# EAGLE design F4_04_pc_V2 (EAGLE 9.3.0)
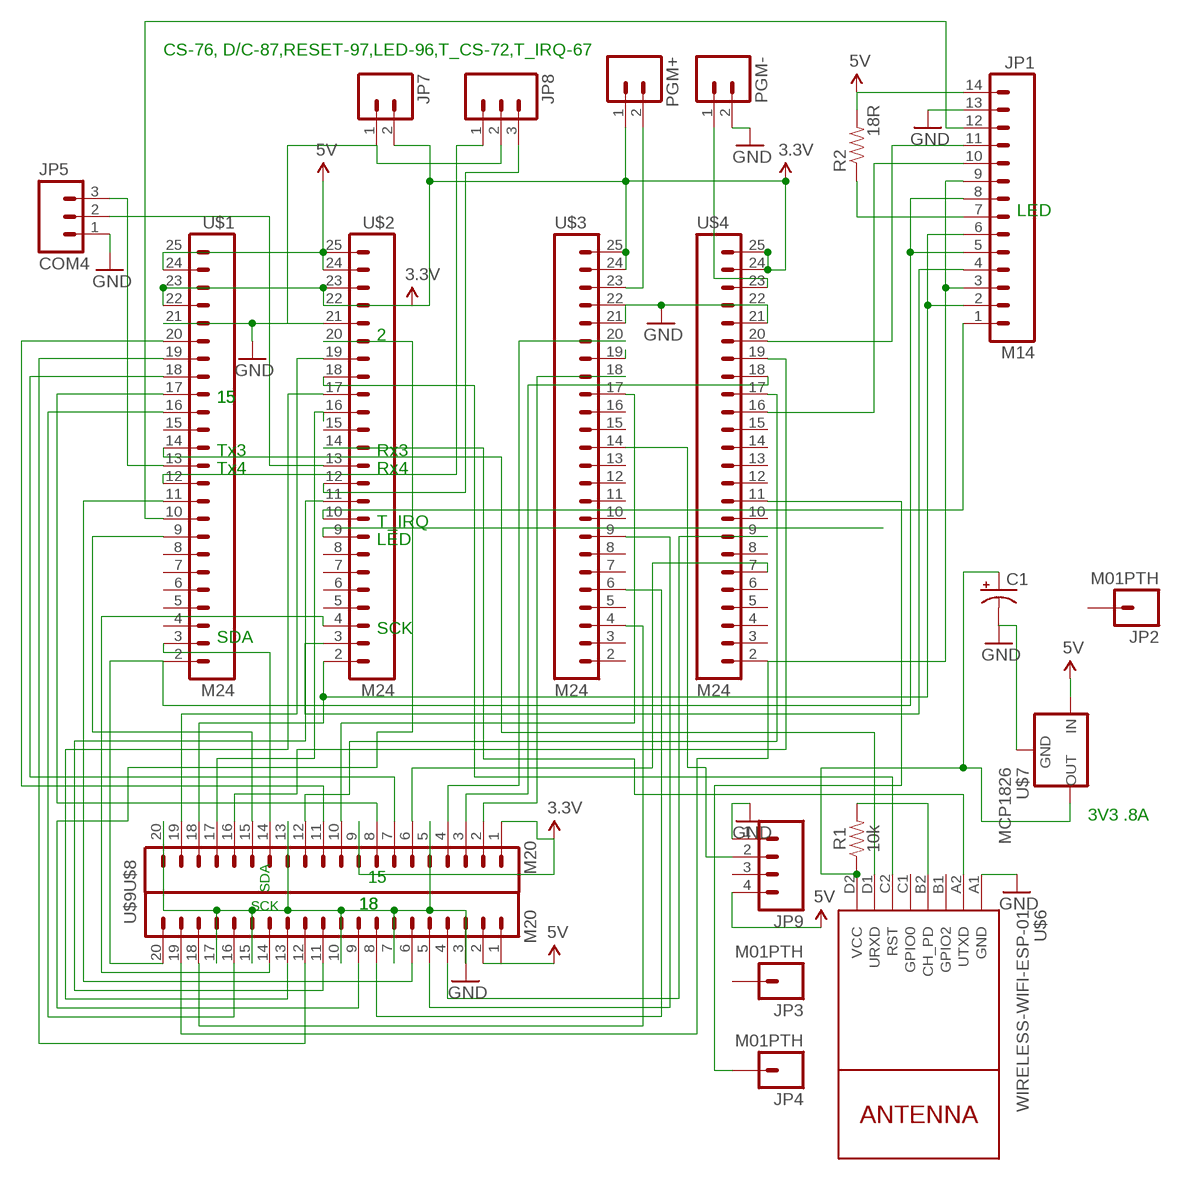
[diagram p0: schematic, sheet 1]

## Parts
C1  CAP_POLD  [PANASONIC_D]
JP1  M14  [1X14]
JP2  M01PTH  [1X01]
JP3  M01PTH  [1X01]
JP4  M01PTH  [1X01]
JP5  COM4  M03PTH  [1X03]
JP7  M02PTH  [1X02]
JP8  M03PTH  [1X03]
JP9  M04LOCK  [1X04_LOCK]
PGM+  M02PTH  [1X02]
PGM-  M02PTH  [1X02]
R1  10k  1KOHM-VERT-1/4W-1%  [AXIAL-0.1]
R2  18R  RESISTORPTH-1/6W  [1/6W-RES]
U$1  M24  [1X24]
U$2  M24  [1X24]
U$3  M24  [1X24]
U$4  M24  [1X24]
U$6  WIRELESS-WIFI-ESP-01  [WIRELESS-WIFI-ESP-01]
U$7  MCP1826  V_REG_MIC2920  [SOT223]
U$8  M20  [1X20]
U$9  M20  [1X20]

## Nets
3.3V: JP7.2 PGM+.1 U$1.22 U$1.23 U$2.22 U$2.23 U$3.24 U$3.25 U$4.24 U$4.25 U$8.1 U$8.9
5V: JP1.14 JP9.4 R2.2 U$1.24 U$1.25 U$2.24 U$2.25 U$7.1(IN) U$9.1 U$9.2
GND: C1.- JP1.13 JP5.1 JP7.1 JP8.2 JP9.1 PGM-.2 U$1.21 U$2.21 U$3.21 U$3.22 U$4.21 U$4.22 U$6.A1(GND) U$7.2(GND) U$8.5 U$8.13 U$8.20 U$9.3 U$9.7 U$9.10 U$9.15 U$9.17
N$1: U$2.9
N$2: U$4.18 U$8.3
N$3: JP1.3 JP1.9 U$4.2 U$9.19
N$4: JP1.2 JP1.6 U$2.2 U$8.18
N$5: JP1.5 JP1.8 U$1.2 U$9.20
N$7: JP1.12 U$1.10
N$8: U$3.18 U$8.2
N$9: JP1.4 U$2.3
N$10: JP1.11 U$4.20
N$11: U$3.20 U$8.4
N$12: U$4.9 U$9.4
N$13: JP1.10 U$4.16
N$14: JP1.1 U$2.10
N$15: U$3.9 U$9.5
N$16: U$3.19
N$17: U$3.6 U$9.8
N$18: U$4.7 U$8.6
N$19: U$2.14 U$6.A2(UTXD)
N$20: U$3.4 U$9.18
N$21: JP9.2 U$3.14
N$22: U$1.14 U$6.D1(URXD)
N$23: JP4.1 U$4.11
N$24: U$2.19 U$8.19
N$25: U$1.9 U$8.15
N$26: U$1.11 U$9.6
N$27: U$2.11 U$9.11
N$28: U$2.17 U$9.13
N$29: U$2.20 U$9.9
N$30: U$1.3 U$8.14
N$31: U$2.4 U$9.14
N$32: U$1.16 U$9.16
N$33: U$3.17 U$8.10
N$34: U$4.17 U$8.12
N$35: U$1.19 U$9.12
N$36: U$1.17 U$8.8
N$37: U$1.18 U$8.7
N$38: U$1.20 U$8.11
N$39: R1.P$2 U$6.B2(CH_PD)
N$40: U$4.19 U$8.16
N$41: U$2.18 U$6.C2(RST)
N$42: PGM+.2 U$3.23
N$43: PGM-.1 U$4.23
N$44: JP1.7 R2.1
N$45: JP8.3 U$2.12
N$46: U$2.16 U$8.17
N$47: JP8.1 U$1.12
N$49: C1.+ R1.P$1 U$6.D2(VCC) U$7.3(OUT)
N$51: JP5.3 U$1.13
N$54: JP5.2 U$2.13
Unconnected: JP2.1 JP3.1 JP9.3 U$1.4 U$1.5 U$1.6 U$1.7 U$1.8 U$1.15 U$2.5 U$2.6 U$2.7 U$2.8 U$2.15 U$3.2 U$3.3 U$3.5 U$3.7 U$3.8 U$3.10 U$3.11 U$3.12 U$3.13 U$3.15 U$3.16 U$4.3 U$4.4 U$4.5 U$4.6 U$4.8 U$4.10 U$4.12 U$4.13 U$4.14 U$4.15 U$6.B1(GPIO2) U$6.C1(GPIO0)

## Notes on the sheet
- CS-76, D/C-87,RESET-97,LED-96,T_CS-72,T_IRQ-67
- LED
- 2
- 15 | 15
- Tx3 | Rx3
- Tx4 | Rx4
- T_IRQ
- LED
- SCK
- SDA
- 3V3 .8A
- 15
- SDA
- SCK
- 18 | 18

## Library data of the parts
C1 = SparkFun-Passives:CAP_POL: Capacitor Polarized
JP1 = 98 SparkFun:M14: Header 14 Standard 14-pin 0.1" header. Use with straight break away headers (SKU : PRT-00116), right angle break away headers (PRT-00553), swiss pins (PRT-00743), machine pins (PRT-00117), and female headers (PRT-00115).
JP2-JP4 = 98 SparkFun:M01: Header 1
JP5 JP8 = 98 SparkFun:M03: Header 3 Standard 3-pin 0.1" header. Use with straight break away headers (SKU : PRT-00116), right angle break away headers (PRT-00553), swiss pins (PRT-00743), machine pins (PRT-00117), and female headers (PRT-00115). Molex polarized connector foot print use with SKU : PRT-08232 with associated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
JP7 PGM+ PGM- = 98 SparkFun:M02: Header 2
JP9 = 98 SparkFun:M04: Header 4 Standard 4-pin 0.1" header. Use with straight break away headers (SKU : PRT-00116), right angle break away headers (PRT-00553), swiss pins (PRT-00743), machine pins (PRT-00117), and female headers (PRT-00115). Molex polarized connector foot print use with SKU : PRT-08231 with associated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
R1 = SparkFun-Resistors:1KOHM: 1kΩ resistor; PROD_ID: RES-12182; VALUE: 1k
R2 = 98 SparkFun:RESISTOR: Resistor
U$1-U$4 = 98 SparkFun:M24
U$6 = 99 diy-modules:WIRELESS-WIFI-ESP-01: Wireless Wi-Fi ESP-01 Module based on ESP8266 chip
U$7 = 98 SparkFun:V_REG_MIC2920: MIC2920A (http://www.micrel.com/_PDF/mic2920.pdf) - 400mA output LDO Regulator
U$8 U$9 = 98 SparkFun:M20: This is just like the LOCK variant in that the holes are staggared by 5 mil, but except for the last two holes. They are not altered from the "standard" footprint layout. This is used for a special purpose on the layout of our Graphic LCD Backpack. Make sure you want to use this device before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

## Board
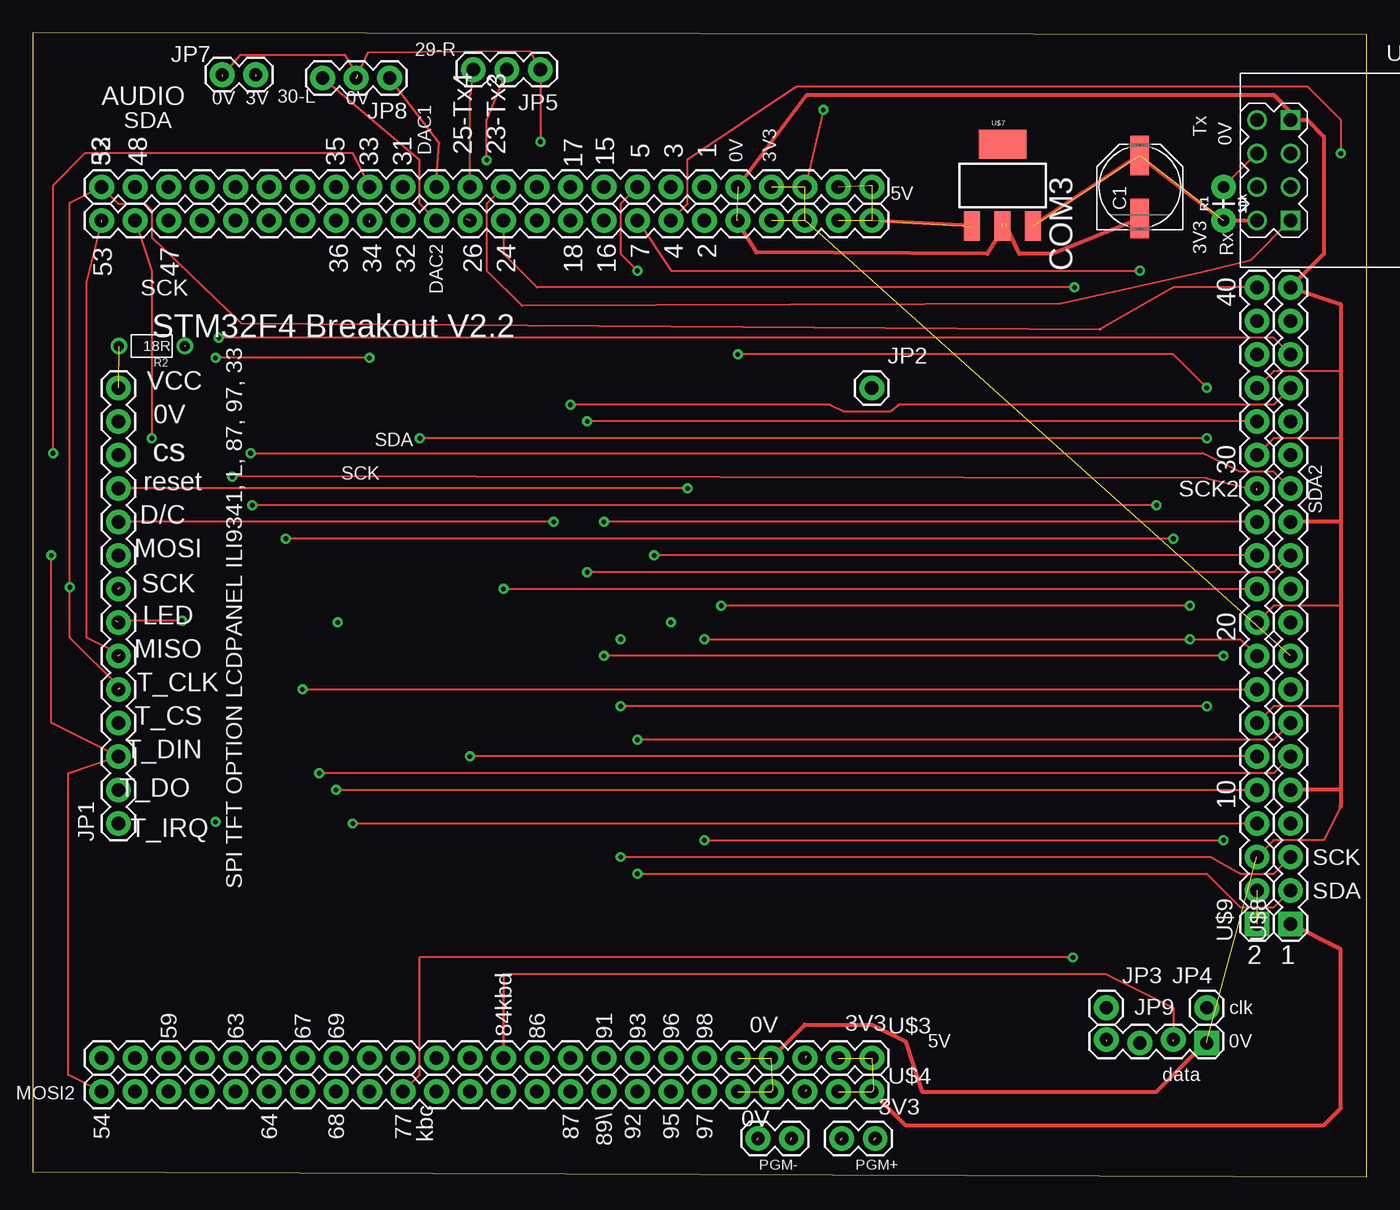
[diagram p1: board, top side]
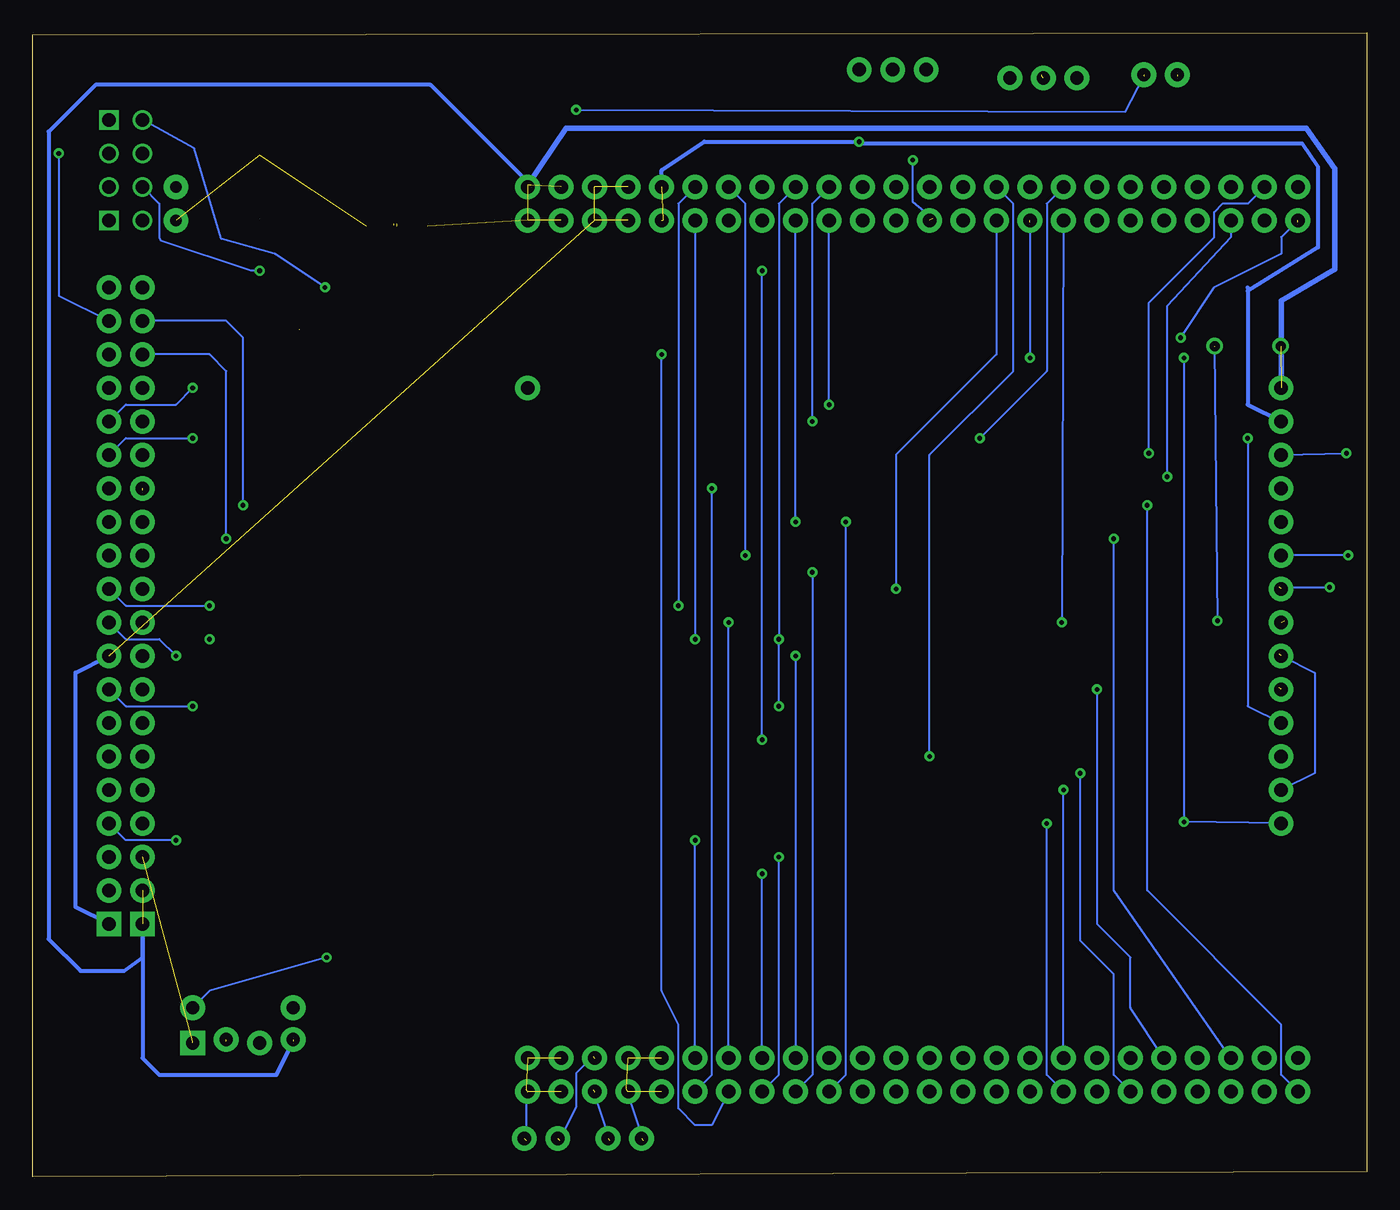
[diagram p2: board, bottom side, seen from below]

Size 101.14 x 86.73 mm. Coordinates in mm from the lower left corner, seen from the top.
Outline: 0,0.38 101.14,0 101.14,86.6 0,86.73 0,0.38
Copper layers (1*16): Top 0.035mm / dielectric 1.5mm / Bottom 0.035mm
Design rules "default": minimum track width 6mil, minimum drill 0.35mm, track to track 6mil, track to pad 6mil, pad to pad 6mil, via to via 6mil, smd to smd 6mil, copper to edge 40mil, drill to drill 6mil, minimum pad ring 10mil, minimum via ring 8mil, stop-mask expansion 4mil, vias tented up to drill 0mil, thermal gap 10mil

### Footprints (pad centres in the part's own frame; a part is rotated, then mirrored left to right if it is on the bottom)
PANASONIC_D = smd 3 x 1.4: + 2.4,0; - -2.4,0
1X14 = drill 1.016 pad 1.88: 1 0,0; 2 2.54,0; 3 5.08,0; 4 7.62,0; 5 10.16,0; 6 12.7,0; 7 15.24,0; 8 17.78,0; 9 20.32,0; 10 22.86,0; 11 25.4,0; 12 27.94,0; 13 30.48,0; 14 33.02,0
1X01 = drill 1.016 pad 1.88: 1 0,0
1X03 = drill 1.016 pad 1.88: 1 0,0; 2 2.54,0; 3 5.08,0
1X02 = drill 1.016 pad 1.88: 1 0,0; 2 2.54,0
1X04_LOCK = drill 1.016 pad 1.88 square: 1 0,0.127 | drill 1.016 pad 1.88: 2 2.54,-0.127; 3 5.08,0.127; 4 7.62,-0.127
AXIAL-0.1 = drill 0.9 pad 1.88: P$1 -1.27,0; P$2 1.27,0
1/6W-RES = drill 0.762: 1 -2.5,0; 2 2.5,0
1X24 = drill 1.016 pad 1.88: 2 -26.67,0; 3 -24.13,0; 4 -21.59,0; 5 -19.05,0; 6 -16.51,0; 7 -13.97,0; 8 -11.43,0; 9 -8.89,0; 10 -6.35,0; 11 -3.81,0; 12 -1.27,0; 13 1.27,0; 14 3.81,0; 15 6.35,0; 16 8.89,0; 17 11.43,0; 18 13.97,0; 19 16.51,0; 20 19.05,0; 21 21.59,0; 22 24.13,0; 23 26.67,0; 24 29.21,0; 25 31.75,0
WIRELESS-WIFI-ESP-01 = drill 1 square: A1 -8.89,3.81; D1 -8.89,-3.81 | drill 1: A2 -11.43,3.81; B1 -8.89,1.27; B2 -11.43,1.27; C1 -8.89,-1.27; C2 -11.43,-1.27; D2 -11.43,-3.81
SOT223 = smd 1.219 x 2.235: 1 -2.311,-3.099; 2 0,-3.099; 3 2.311,-3.099 | smd 3.6 x 2.2: 4 0,3.099
1X20 = drill 1.016 pad 1.88 square: 1 0,0 | drill 1.016 pad 1.88: 2 2.54,0; 3 5.08,0; 4 7.62,0; 5 10.16,0; 6 12.7,0; 7 15.24,0; 8 17.78,0; 9 20.32,0; 10 22.86,0; 11 25.4,0; 12 27.94,0; 13 30.48,0; 14 33.02,0; 15 35.56,0; 16 38.1,0; 17 40.64,0; 18 43.18,0; 19 45.72,0; 20 48.26,0

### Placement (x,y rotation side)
C1  83.95,75.06 90 top
JP1  6.48,26.8 90 top
JP2  63.63,59.82 0 top
JP3  81.41,12.83 0 top
JP4  89.03,12.83 0 top
JP5  38.48,83.95 180 top
JP7  14.35,83.57 0 top
JP8  27.05,83.31 180 top
JP9  89.03,10.29 180 top
PGM+  63.88,2.92 180 top
PGM-  57.53,2.92 180 top
R1  90.3,73.79 90 top
R2  9.02,62.99 180 top
U$1  31.88,75.06 0 top
U$2  31.88,72.52 0 top
U$3  31.88,9.02 0 top
U$4  31.88,6.48 0 top
U$6  104.27,76.33 0 top
U$7  73.53,75.18 0 top
U$8  95.38,19.18 90 top
U$9  92.84,19.18 90 top

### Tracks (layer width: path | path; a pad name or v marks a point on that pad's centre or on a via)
3.3V  (via drill 0.35)  (11 unrouted)
  Top 0.152: v59.94,80.9 58.55,74.93
  Top 0.305: U$4.25 66.17,3.94 97.92,3.94 99.19,5.21 99.19,17.27 U$8.1
  Bottom 0.152: 63.75,6.6 63.75,2.79 | v59.94,80.9 18.29,80.77 16.89,83.44
  Bottom 0.305: U$8.1 97.92,20.45 97.92,38.23 U$8.9
5V  (9 unrouted)
  Bottom 0.305: 81.41,10.29 82.68,7.75 91.57,7.75 92.84,9.02 U$9.1 92.84,16.64 94.23,15.62 97.54,15.62 99.95,18.03 99.95,79.25 96.39,82.8 70.99,82.8 63.37,75.18
  Bottom 0.406: JP1.14 6.48,66.42 2.41,68.83 2.41,76.45 4.57,79.5 60.71,79.5 63.63,75.18
GND  (via drill 0.35)  (15 unrouted)
  Top 0.152: 99.19,61.09 94.11,61.09 U$9.17 | 99.19,56.01 94.11,56.01 U$9.15 | 99.19,43.31 94.11,43.31 U$9.10 | 99.19,35.69 94.11,35.69 U$9.7 | 99.19,28.07 97.92,25.53 94.11,25.53 U$9.3 | v38.48,78.49 JP5.1 37.72,85.34 25.4,85.22 24.64,83.57 | 14.35,83.44 15.75,85.09 23.62,85.09 24.64,83.44
  Top 0.305: 53.47,75.69 U$1.21 58.71,82.04 94.11,82.04 95.38,80.77 U$6.A1 96.65,80.14 97.92,78.87 97.92,69.98 U$8.20 99.19,66.17 99.19,61.09 99.19,56.01 99.19,49.66 | 99.19,49.66 99.19,43.31 99.19,35.69 99.19,29.34 | 99.19,29.34 99.19,28.07 | 99.19,49.66 U$8.13 | 99.19,29.34 U$8.5 | U$3.22 58.55,11.56 63.63,11.56 66.17,10.29 67.44,6.48 85.22,6.48 89.03,10.29 | 73.53,72.26 73.79,72.26 72.39,69.98 54.86,70.1 53.34,72.52 | C1.- 77.34,69.98 74.8,69.98 73.79,72.14
  Bottom 0.152: 56.13,6.6 54.86,2.79
  Bottom 0.305: U$1.21 53.47,76.33 50.23,78.49 v38.48,78.49 38.35,78.36 4.9,78.36 3.68,76.58 3.68,70.48 9.02,67.18 | 9.02,67.44 9.02,67.18 | 9.02,67.18 9.02,58.55 JP1.13 | 95.38,67.56 U$8.20
N$1  (via drill 0.35)
  Bottom 0.152: U$2.9 v23.11,42.04
N$2  (via drill 0.35)
  Top 0.152: v44.58,24.26 89.28,24.26 91.57,22.99 94.11,22.99 U$8.3
  Bottom 0.152: U$4.18 44.58,7.75 v44.58,24.26
N$3  (via drill 0.35)
  Top 0.152: U$4.2 2.67,7.75 2.67,30.61 JP1.3 1.4,34.42 v1.4,47.12 | v85.22,50.93 v16.64,50.93
  Bottom 0.152: v1.4,47.12 JP1.9 | U$4.2 6.48,7.75 6.48,11.56 16.64,21.72 v16.64,50.93 | v85.22,50.93 85.22,63.63 86.49,64.9 U$9.19
N$4  (via drill 0.35)  (2 unrouted)
  Top 0.152: U$8.18 94.11,63.63 v14.1,63.63 | 6.6,39.62 4.06,40.89 4.06,67.82 5.21,72.39
  Bottom 0.152: JP1.6 3.94,38.23 3.94,30.61 JP1.2 | U$2.2 6.48,71.25 6.48,69.98 11.56,67.44 v14.1,63.63
N$5  (via drill 0.35)  (3 unrouted)
  Top 0.152: 80.97,64.26 15.8,64.71 9.02,71.25 9.02,73.28 8.51,73.79 6.48,73.79 U$1.2 2.79,73.85 v2.79,44.7 2.79,40.89 6.6,37.08 | U$9.20 86.49,67.44 80.9,64.26
  Bottom 0.152: 6.6,44.7 v2.79,44.7
N$6  (via drill 0.35)
  other vias: 13.84,26.92
N$7  (via drill 0.35)
  Top 0.152: U$1.10 24.26,77.6 3.94,77.6 1.52,75.18 v1.52,54.86
  Bottom 0.152: 6.35,54.86 JP1.12 v1.52,54.86
N$8  (via drill 0.35)
  Top 0.152: v45.85,22.99 89.03,22.99 91.57,20.45 94.11,20.45 U$8.2
  Bottom 0.152: U$3.18 v45.85,22.99
N$9  (via drill 0.35)
  Top 0.152: U$2.3 9.02,68.71 v9.02,56.01
  Bottom 0.152: v9.02,56.01 9.02,35.69 JP1.4
N$10  (via drill 0.35)
  Top 0.152: v49.66,52.2 JP1.11
  Bottom 0.152: U$4.20 49.66,7.75 v49.66,52.2
N$11  (via drill 0.35)
  Top 0.152: v50.93,25.53 v90.3,25.53
  Bottom 0.152: U$3.20 v50.93,25.53 | v90.3,25.53 94.11,25.53 U$8.4
N$12  (via drill 0.35)
  Top 0.152: v24.26,26.8 U$9.4
  Bottom 0.152: U$4.9 24.26,7.75 v24.26,26.8
N$13  (via drill 0.35)
  Top 0.152: v39.5,49.66 JP1.10
  Bottom 0.152: U$4.16 39.5,7.75 v39.5,49.66
N$14  (via drill 0.35)  (1 unrouted)
  Top 0.152: v25.53,62.1 v13.84,62.1 13.72,62.1
  Bottom 0.152: 25.53,72.39 v25.53,62.1 | v13.84,62.1 13.84,26.92 JP1.1
N$15  (via drill 0.35)
  Top 0.152: v22.99,29.34 U$9.5
  Bottom 0.152: U$3.9 v22.99,29.34
N$16  (via drill 0.35)
  Bottom 0.152: U$3.19 v48.39,42.04
N$17  (via drill 0.35)
  Top 0.152: v20.45,36.96 U$9.8
  Bottom 0.152: U$3.6 17.91,12.83 17.91,16.64 20.45,19.18 v20.45,36.96
N$18  (via drill 0.35)
  Top 0.152: U$8.6 94.11,30.61 v21.72,30.61
  Bottom 0.152: U$4.7 19.18,7.75 19.18,15.37 21.72,17.91 v21.72,30.61
N$19  (via drill 0.35)
  Top 0.152: U$2.14 35.69,69.98 38.23,67.44 v78.99,67.44 79.12,67.44
  Bottom 0.152: v78.99,67.44 82.8,69.98 86.87,71.12 88.9,77.98 U$6.A2
N$20  (via drill 0.35)
  Top 0.152: v86.49,48.39 v19.18,48.39
  Bottom 0.152: U$3.4 19.18,21.72 v19.18,48.39 | v86.49,48.39 86.49,61.09 87.76,62.36 U$9.18
N$21  (1 unrouted)
  Top 0.152: 35.69,14.1 U$3.14 35.69,15.37 81.41,15.37 86.49,12.83 86.49,10.29
N$22
  Top 0.152: U$1.14 34.42,73.79 34.42,68.71 37.08,66.04 77.79,66.21 89.03,68.71 92.41,69.55 U$6.D1
N$23  (via drill 0.35)
  Top 0.152: U$4.11 29.34,7.75 29.34,16.64 v78.87,16.64
  Bottom 0.152: v78.87,16.64 87.76,14.1 JP4.1
N$24  (via drill 0.35)
  Top 0.152: U$2.19 49.66,73.79 49.66,77.17 57.91,82.68 96.65,82.68 99.19,80.14 v99.19,77.6
  Bottom 0.152: v99.19,77.6 99.19,66.8 U$8.19
N$25  (via drill 0.35)
  Top 0.152: v89.03,56.01 v29.34,56.01
  Bottom 0.152: U$8.15 94.11,56.01 v89.03,56.01 | U$1.9 24.26,73.79 24.26,61.09 v29.34,56.01
N$26  (via drill 0.35)
  Top 0.152: U$9.6 v33.15,31.88
  Bottom 0.152: v33.15,31.88 33.15,54.74 26.8,61.09 26.8,73.79 U$1.11
N$27  (via drill 0.35)
  Top 0.152: v35.69,44.58 U$9.11
  Bottom 0.152: U$2.11 28.07,62.36 35.69,54.74 v35.69,44.58
N$28  (via drill 0.35)
  Top 0.152: U$9.13 v43.31,49.66
  Bottom 0.152: v43.31,49.66 U$2.17
N$29  (via drill 0.35)
  Top 0.152: U$9.9 91.57,40.77 v87.76,40.77 v50.93,40.77
  Bottom 0.152: U$2.20 v50.93,40.77
N$30  (via drill 0.35)
  Top 0.152: U$8.14 94.11,53.47 91.57,53.47 88.77,54.86 v16.51,54.86
  Bottom 0.152: U$1.3 9.02,73.79 10.92,73.79 11.56,73.15 11.56,71.25 16.51,66.29 v16.51,54.86
N$31  (via drill 0.35)  (1 unrouted)
  Top 0.152: v15.11,53.09 15.17,53.14 89.03,52.96 92.84,52.07
  Bottom 0.152: U$2.4 10.29,71.25 15.11,66.04 v15.11,53.09
N$32  (via drill 0.35)
  Top 0.152: U$9.16 v42.04,57.28
  Bottom 0.152: v42.04,57.28 42.04,73.79 U$1.16
N$33  (via drill 0.35)
  Top 0.152: v90.3,39.5 v43.31,39.5
  Bottom 0.152: U$8.10 94.11,40.77 91.57,40.77 v90.3,39.5 | v43.31,39.5 U$3.17
N$34  (via drill 0.35)
  Top 0.152: U$8.12 94.11,45.85 v42.04,45.85
  Bottom 0.152: v42.04,45.85 42.04,7.75 U$4.17
N$35  (via drill 0.35)
  Top 0.152: U$9.12 v47.12,47.12
  Bottom 0.152: v47.12,47.12 47.12,73.79 U$1.19
N$36  (via drill 0.35)
  Top 0.152: v89.03,35.69 v44.58,35.69
  Bottom 0.152: U$8.8 94.11,35.69 v89.03,35.69 | U$1.17 44.58,73.79 v44.58,40.77 v44.58,35.69
N$37  (via drill 0.35)
  Top 0.152: U$8.7 94.11,33.15 v45.85,33.15 | U$1.18 44.58,73.79 44.58,69.98 v45.85,68.71
  Bottom 0.152: v45.85,33.15 v45.85,68.71
N$38  (via drill 0.35)
  Top 0.152: v87.76,43.31 v52.2,43.31
  Bottom 0.152: U$1.20 52.2,73.79 v52.2,43.31 | U$8.11 94.11,43.31 v87.76,43.31
N$39
  Top 0.152: U$6.B2 R1.P$2
N$40  (via drill 0.35)
  Top 0.152: v89.03,59.82 86.49,62.36 v53.47,62.36
  Bottom 0.152: U$4.19 49.66,3.94 50.93,3.94 52.2,5.21 52.2,11.56 53.47,14.1 v53.47,62.36 | U$8.16 94.11,58.55 90.3,58.55 v89.03,59.82
N$41  (via drill 0.35)
  Top 0.152: U$2.18 48.39,68.71 v83.95,68.71
  Bottom 0.152: v83.95,68.71 84.58,68.71 91.44,70.99 91.57,71.25 91.57,73.79 U$6.C2
N$42  (2 unrouted)
  Bottom 0.152: 58.67,9.14 59.94,7.87 59.94,5.33 61.21,2.79
N$43  (2 unrouted)
  Bottom 0.152: 58.67,6.6 57.4,2.79
N$44  (via drill 0.35)  (2 unrouted)
  Top 0.152: v11.3,42.16 6.22,42.16
  Bottom 0.152: 11.56,62.99 v11.3,42.16
N$45
  Top 0.152: U$2.12 29.34,73.79 29.34,77.08 JP8.3
N$46  (via drill 0.35)
  Top 0.152: U$8.17 94.11,58.55 65.66,58.55 65.02,58.04 61.47,58.04 60.45,58.55 v40.77,58.55
  Bottom 0.152: v40.77,58.55 U$2.16
N$47
  Top 0.152: U$1.12 30.61,75.69 30.6,75.7 30.81,78.4 JP8.1
N$49  (2 unrouted)
  Top 0.305: R1.P$1 U$6.D2
N$50
  Top 0.305: 63.75,72.52 71.25,72.14
N$51
  Top 0.152: JP5.3 33.15,82.01 U$1.13
N$52
  Top 0.305: 76.07,72.64 75.82,72.14 83.82,77.47 90.42,72.39
N$54  (via drill 0.35)  (1 unrouted)
  Top 0.152: JP5.2 34.42,80.14 v34.42,77.09
  Bottom 0.152: 32.89,72.64 34.42,73.91 v34.42,77.09

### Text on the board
_tsilk: 29-R | 25-Tx4 | 23-Tx3 | AUDIO | 0V | 3V | 30-L | 0V | DAC1 | 33 | 52 | SDA | 48 | 35 | 33 | 31 | 15 | Tx | 17 | 5 | 3 | 1 | 0V | 0V | 3V3 | 5V | 53 | 47 | 36 | 34 | 32 | DAC2 | 26 | 24 | 18 | 16 | 7 | 4 | 2 | 3V3 | Rx | COM3 | 40 | SCK | STM32F4 Breakout V2.2 | VCC | 0V | cs | SDA | 30 | reset | SCK | D/C | SCK2 | SDA2 | MOSI | SCK | LED | 20 | MISO | T_CLK | T_CS | T_DIN | T_DO | 10 | T_IRQ | SCK | SPI TFT OPTION LCDPANEL ILI9341, L, 87, 97, 33 | SDA | 2 | 1 | 84kbd | 59 | 63 | 67 | 69 | 86 | 91 | 93 | 96 | 98 | clk | 0V | 3V3 | 5V | 0V | MOSI2 | data | 54 | 64 | 68 | 77 | kbc | 87 | 89\ | 92 | 95 | 97 | 0V | 3V3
